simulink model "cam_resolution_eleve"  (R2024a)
settings: Solver=VariableStepAuto  StartTime=0.0  StopTime=10.0  RelTol=1e-3
model workspace (MAT data in the model file):
  distance = 10
  w_s_exp = 90

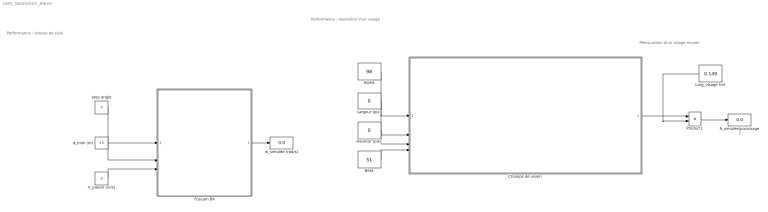
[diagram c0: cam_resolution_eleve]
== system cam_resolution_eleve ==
  note: Mensuration d'un visage moyen
  note: Performance : vitesse de suivi
  note: Performance : resolution d'un visage
  Alpha : Constant  Value=98
  Beta : Constant  Value=51
  Champs de vision : Subsystem
  Foscam B4 : Subsystem
  Hauteur (pix) : Constant  Value=0
  Larg_visage (m) : Constant  Value=0.149
  Largeur (pix) : Constant  Value=0
  Product1 : Product
  R_simulée(pix/visage) : Display
  V_pieton (m/s) : Constant  Value=0
  d_mini (m) : Constant  Value=3.5
  step angle : Constant  Value=0
  w_simulée (rad/s) : Display
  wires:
  Product1/1 -> R_simulée(pix/visage)/1
  Larg_visage (m)/1 -> Product1/2
  Alpha/1 -> Champs de vision/1(alpha)
  Largeur (pix)/1 -> Champs de vision/2(In2)
  Hauteur (pix)/1 -> Champs de vision/3(In3)
  Beta/1 -> Champs de vision/4(beta)
  Champs de vision/1(Out1) -> Product1/1
  d_mini (m)/1 -> Foscam B4/2(In2)
  V_pieton (m/s)/1 -> Foscam B4/3(In3)
  Foscam B4/1(Out1) -> w_simulée (rad/s)/1
  step angle/1 -> Foscam B4/1(In1)

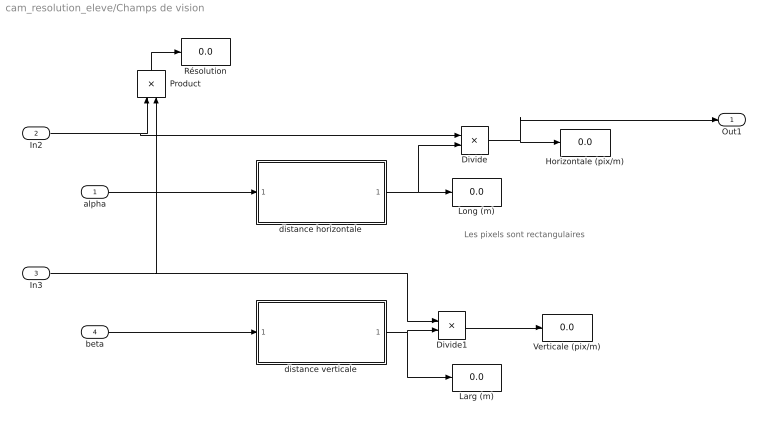
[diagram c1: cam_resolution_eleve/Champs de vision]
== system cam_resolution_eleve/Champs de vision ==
  note: Les pixels sont rectangulaires
  alpha : Inport
  In2 : Inport  Port=2
  In3 : Inport  Port=3
  beta : Inport  Port=4
  Divide : Product  Inputs=*/
  Divide1 : Product  Inputs=*/
  Horizontale (pix/m) : Display
  Larg (m) : Display
  Long (m) : Display
  Product : Product
  Résolution : Display
  Verticale (pix/m) : Display
  distance horizontale : MATLAB Function  TreatAsAtomicUnit=on
  distance verticale : MATLAB Function  TreatAsAtomicUnit=on
  Out1 : Outport
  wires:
  alpha/1 -> distance horizontale/1(alpha)
  distance verticale/1(Larg) -> Divide1/2, Larg (m)/1
  Product/1 -> Résolution/1
  distance horizontale/1(Long) -> Long (m)/1, Divide/2
  In2/1 -> Product/1, Divide/1
  Divide/1 -> Out1/1, Horizontale (pix/m)/1
  beta/1 -> distance verticale/1(beta)
  In3/1 -> Divide1/1, Product/2
  Divide1/1 -> Verticale (pix/m)/1

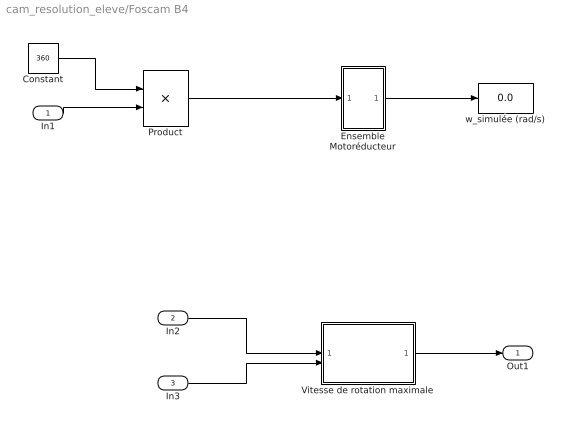
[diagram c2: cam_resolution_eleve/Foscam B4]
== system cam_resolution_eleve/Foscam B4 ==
  In1 : Inport
  In2 : Inport  Port=2
  In3 : Inport  Port=3
  Constant : Constant  Value=360
  Ensemble Motoréducteur : Subsystem
  Product : Product  Inputs=*/
  Vitesse de rotation maximale : MATLAB Function  TreatAsAtomicUnit=on
  w_simulée (rad/s) : Display
  Out1 : Outport  VectorParamsAs1DForOutWhenUnconnected=off
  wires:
  Ensemble Motoréducteur/1(w_s) -> w_simulée (rad/s)/1
  In2/1 -> Vitesse de rotation maximale/1(d_mini)
  Vitesse de rotation maximale/1(w_max) -> Out1/1
  In3/1 -> Vitesse de rotation maximale/2(V_pieton)
  Product/1 -> Ensemble Motoréducteur/1(s)
  In1/1 -> Product/2
  Constant/1 -> Product/1

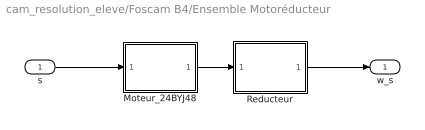
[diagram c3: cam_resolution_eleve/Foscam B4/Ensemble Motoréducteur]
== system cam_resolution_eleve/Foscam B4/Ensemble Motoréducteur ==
  s : Inport
  Moteur_24BYJ48 : MATLAB Function  TreatAsAtomicUnit=on
  Reducteur : MATLAB Function  TreatAsAtomicUnit=on
  w_s : Outport
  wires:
  Moteur_24BYJ48/1(w_m) -> Reducteur/1(w_e)
  s/1 -> Moteur_24BYJ48/1(s)
  Reducteur/1(w_s) -> w_s/1

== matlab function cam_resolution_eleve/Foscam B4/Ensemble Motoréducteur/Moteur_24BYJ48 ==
function w_m = fcn(s)

stepper = 360/s; %résultat en °/pas
w = 4.08; %tr/s
w_m = w*(2*pi); %résultat en rad/s

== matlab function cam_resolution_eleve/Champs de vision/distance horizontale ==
function Long = fcn(alpha)

distance  = 6;

Long = 2*distance*tan((alpha*(pi/180))/2);

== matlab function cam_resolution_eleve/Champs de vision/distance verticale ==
function Larg = fcn(beta)

distance  = 6;

Larg = 2*distance*tan(beta*(pi/180)/2);

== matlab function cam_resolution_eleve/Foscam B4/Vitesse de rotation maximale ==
function w_max = fcn(d_mini,V_pieton)

w_max = V_pieton/d_mini;

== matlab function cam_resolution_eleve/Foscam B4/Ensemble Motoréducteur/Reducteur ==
function w_s = fcn(w_e)

r = 1/64; %rapport de transmission
w_s = (w_e*r);
